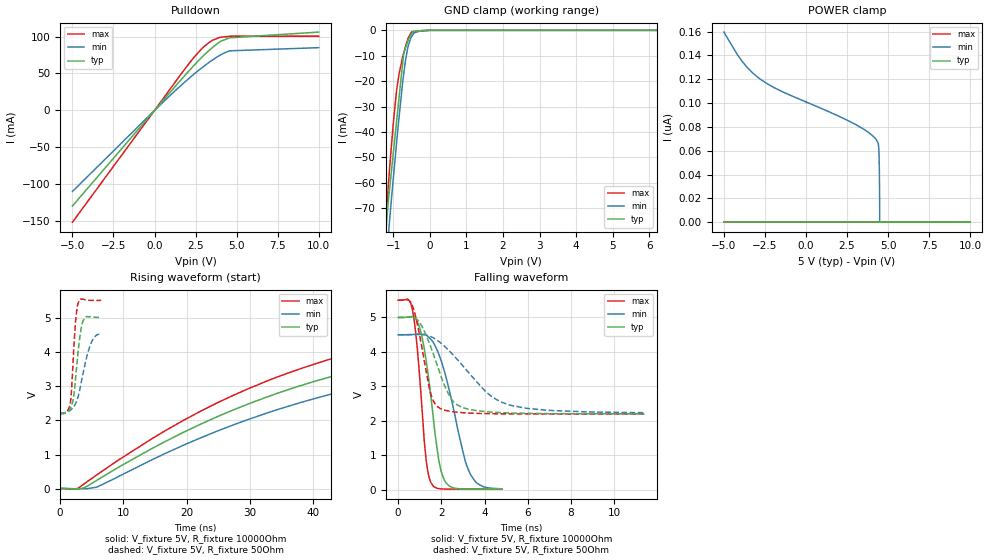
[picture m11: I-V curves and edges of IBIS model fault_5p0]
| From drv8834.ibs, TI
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|   fault_5p0 Model
[Model]   fault_5p0
Model_type   Open_drain
Polarity   Inverting
Vmeas = 2.5
Vref = 5
Cref = 2pF
Rref = 10000
|   typ   min   max
|   (nom PVT)   (fast PVT)   (slow PVT)
|C_comp from frequency sweep method (F = 125KHz)
|C_comp   1.075e-10   7.072e-11   8.192e-10
|ON state : BUFFER OUTPUT TURNED LOW
|C_comp   1.075e-10   7.072e-11   8.192e-10
|OFF state: BUFFER IN HIGH IMPEDANCE
|C_comp   3.510e-12   3.285e-12   3.744e-12
|C_comp from LC tank measurement(L=1nH)
|Resonant Frequency(Hz)   4.050e+09   4.060e+09   3.900e+09
 C_comp   1.546e-12   1.538e-12   1.667e-12
|ON state : BUFFER OUTPUT TURNED LOW
|Resonant Frequency(Hz)   4.050e+09   4.060e+09   3.900e+09
|C_comp   1.546e-12   1.538e-12   1.667e-12
|OFF state: BUFFER IN HIGH IMPEDANCE
|Resonant Frequency(Hz)   3.310e+09   3.370e+09   3.240e+09
|C_comp   2.314e-12   2.233e-12   2.415e-12
| Where nom  PVT is Nominal Process, 5V, 27C
|   Fast PVT is Strong Process,  5.5V, -40C
|   Slow PVT is Weak Process,   4.5V, 125C
[Voltage Range]   5   4.5   5.5
|Ambient Temperature   25   150   -40
|Junction Temperature
[Temperature Range]   27   125   -40
[Pullup Reference]   5   4.5   5.5
[Pulldown Reference]   0   0   0
[Power Clamp Reference]   5   4.5   5.5
[GND Clamp Reference]   0   0   0
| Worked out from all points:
|   slope of the pulldown table from 0 to 0.75 V, typ, clamps not added: 38.7 ohm
|   GND clamp passes 1 mA (typ) near -0.48 V on its own axis
|   falling waveform, V_fixture 5V, R_fixture 10000Ohm: 20-80 % time 612ps typ, 1.01ns min, 417ps max; typ from 5 V to 0.022 V
|   rising waveform, V_fixture 5V, R_fixture 10000Ohm: 20-80 % time 47.5ns typ, 50.1ns min, 44.5ns max; typ from 0.019 V to 4.98 V
|   falling waveform, V_fixture 5V, R_fixture 50Ohm: 20-80 % time 1.02ns typ, 2.04ns min, 600ps max; typ from 5 V to 2.21 V
|   rising waveform, V_fixture 5V, R_fixture 50Ohm: 20-80 % time 935ps typ, 1.7ns min, 634ps max; typ from 2.2 V to 5 V
[Pulldown]
|   Voltage   I(typ)   I(min)   I(max)
-5V       -129.3mA   -109.6mA   -151.2mA
733.5mV   18.97mA    15.77mA    22.32mA
2.272V    57.73mA    46.68mA    68.31mA
2.882V    71.9mA     57.6mA     83.61mA
3.41V     82.9mA     66.53mA    93.22mA
4.035V    93.61mA    75.23mA    98.95mA
4.582V    98.3mA     80.67mA    100.4mA
10V       106mA      84.93mA    100.4mA
[GND Clamp]
|   Voltage   I(typ)   I(min)   I(max)
-5V       -849.5mA   -864.5mA   -886.5mA
-1.373V   -111.3mA   -121.9mA   -108.4mA
-1.14V    -68.15mA   -82.05mA   -62.52mA
-1.095V   -61.85mA   -74.25mA   -53.54mA
-995.5mV  -48.15mA   -58.09mA   -36.46mA
-902mV    -35.21mA   -43.61mA   -23.14mA
-836mV    -26.08mA   -33.75mA   -16.91mA
-715mV    -9.331mA   -17.58mA   -9.057mA
-603mV    -4.488mA   -6.957mA   -3.586mA
-495mV    -1.194mA   -2.394mA   -582.4uA
-202.5mV  -179.2uA   -12.65uA   -238.3uA
10V       0A         0A         0A
[POWER Clamp]
|   Voltage   I(typ)   I(min)   I(max)
-5V       0A         159.6nA    0A
-3.888V   0A         135nA      0A
-2.83V    0A         120.6nA    0A
3.06V     0A         81.75nA    0A
4.253V    0A         69.85nA    0A
4.396V    0A         66.18nA    0A
4.446V    0A         59.82nA    0A
4.464V    0A         50.79nA    0A
4.478V    0A         37.77nA    0A
4.491V    0A         17.72nA    0A
4.495V    0A         0A         0A
10V       0A         0A         0A
[Ramp]
R_load = 10000
|   typ   min   max
dV/dt_r   2.98853/4.8108e-08   2.68712/5.10059e-08   3.28919/4.48666e-08
dV/dt_f   2.98853/6.12395e-10   2.68712/1.00999e-09   3.28919/4.1755e-10
[Falling Waveform]
V_fixture = 5V
V_fixture_min = 4.5V
V_fixture_max = 5.5V
R_fixture = 10000Ohm
C_fixture = 0F
|   Time   V(typ)   V(min)   V(max)
0s        5V         4.499V     5.5V
475ps     5.015V     4.5V       5.518V
700ps     5.01V      4.507V     5.083V
925ps     4.823V     4.516V     3.82V
1.275ns   3.835V     4.494V     992.3mV
1.525ns   2.652V     4.359V     199.5mV
1.875ns   884.3mV    3.945V     36.65mV
2.2ns     216.6mV    3.304V     21.23mV
3.325ns   21.93mV    476.6mV    21.69mV
4.8ns     22.4mV     28.36mV    18.65mV
[Rising Waveform]
V_fixture = 5V
V_fixture_min = 4.5V
V_fixture_max = 5.5V
R_fixture = 10000Ohm
C_fixture = 0F
|   Time   V(typ)   V(min)   V(max)
0s        19.11mV    20.46mV    18.01mV
2.825ns   3.746mV    9.48mV     24.28mV
5.775ns   252.7mV    54.76mV    411.9mV
19.53ns   1.657V     1.281V     2.006V
32.8ns    2.691V     2.223V     3.158V
45.58ns   3.412V     2.893V     3.94V
60.2ns    3.981V     3.436V     4.535V
77.53ns   4.404V     3.852V     4.963V
102.4ns   4.726V     4.184V     5.27V
178.9ns   4.976V     4.466V     5.483V
[Falling Waveform]
V_fixture = 5V
V_fixture_min = 4.5V
V_fixture_max = 5.5V
R_fixture = 50Ohm
C_fixture = 0F
|   Time   V(typ)   V(min)   V(max)
0s        5V         4.5V       5.5V
450ps     5.006V     4.5V       5.513V
675ps     5.004V     4.503V     5.311V
1.05ns    4.798V     4.504V     4.295V
1.475ns   4.202V     4.455V     2.862V
1.95ns    3.358V     4.27V      2.358V
2.725ns   2.467V     3.789V     2.252V
4.05ns    2.268V     2.849V     2.211V
5.075ns   2.232V     2.475V     2.204V
11.4ns    2.206V     2.237V     2.199V
[Rising Waveform]
V_fixture = 5V
V_fixture_min = 4.5V
V_fixture_max = 5.5V
R_fixture = 50Ohm
C_fixture = 0F
|   Time   V(typ)   V(min)   V(max)
0s        2.2V       2.217V     2.193V
1.1ns     2.251V     2.242V     2.266V
1.625ns   2.362V     2.298V     2.543V
2.05ns    2.597V     2.376V     3.735V
2.4ns     3.142V     2.474V     4.794V
2.85ns    4.027V     2.697V     5.426V
3.35ns    4.708V     3.134V     5.53V
3.975ns   5.002V     3.677V     5.516V
5.025ns   5.014V     4.31V      5.499V
6.5ns     4.999V     4.516V     5.5V
